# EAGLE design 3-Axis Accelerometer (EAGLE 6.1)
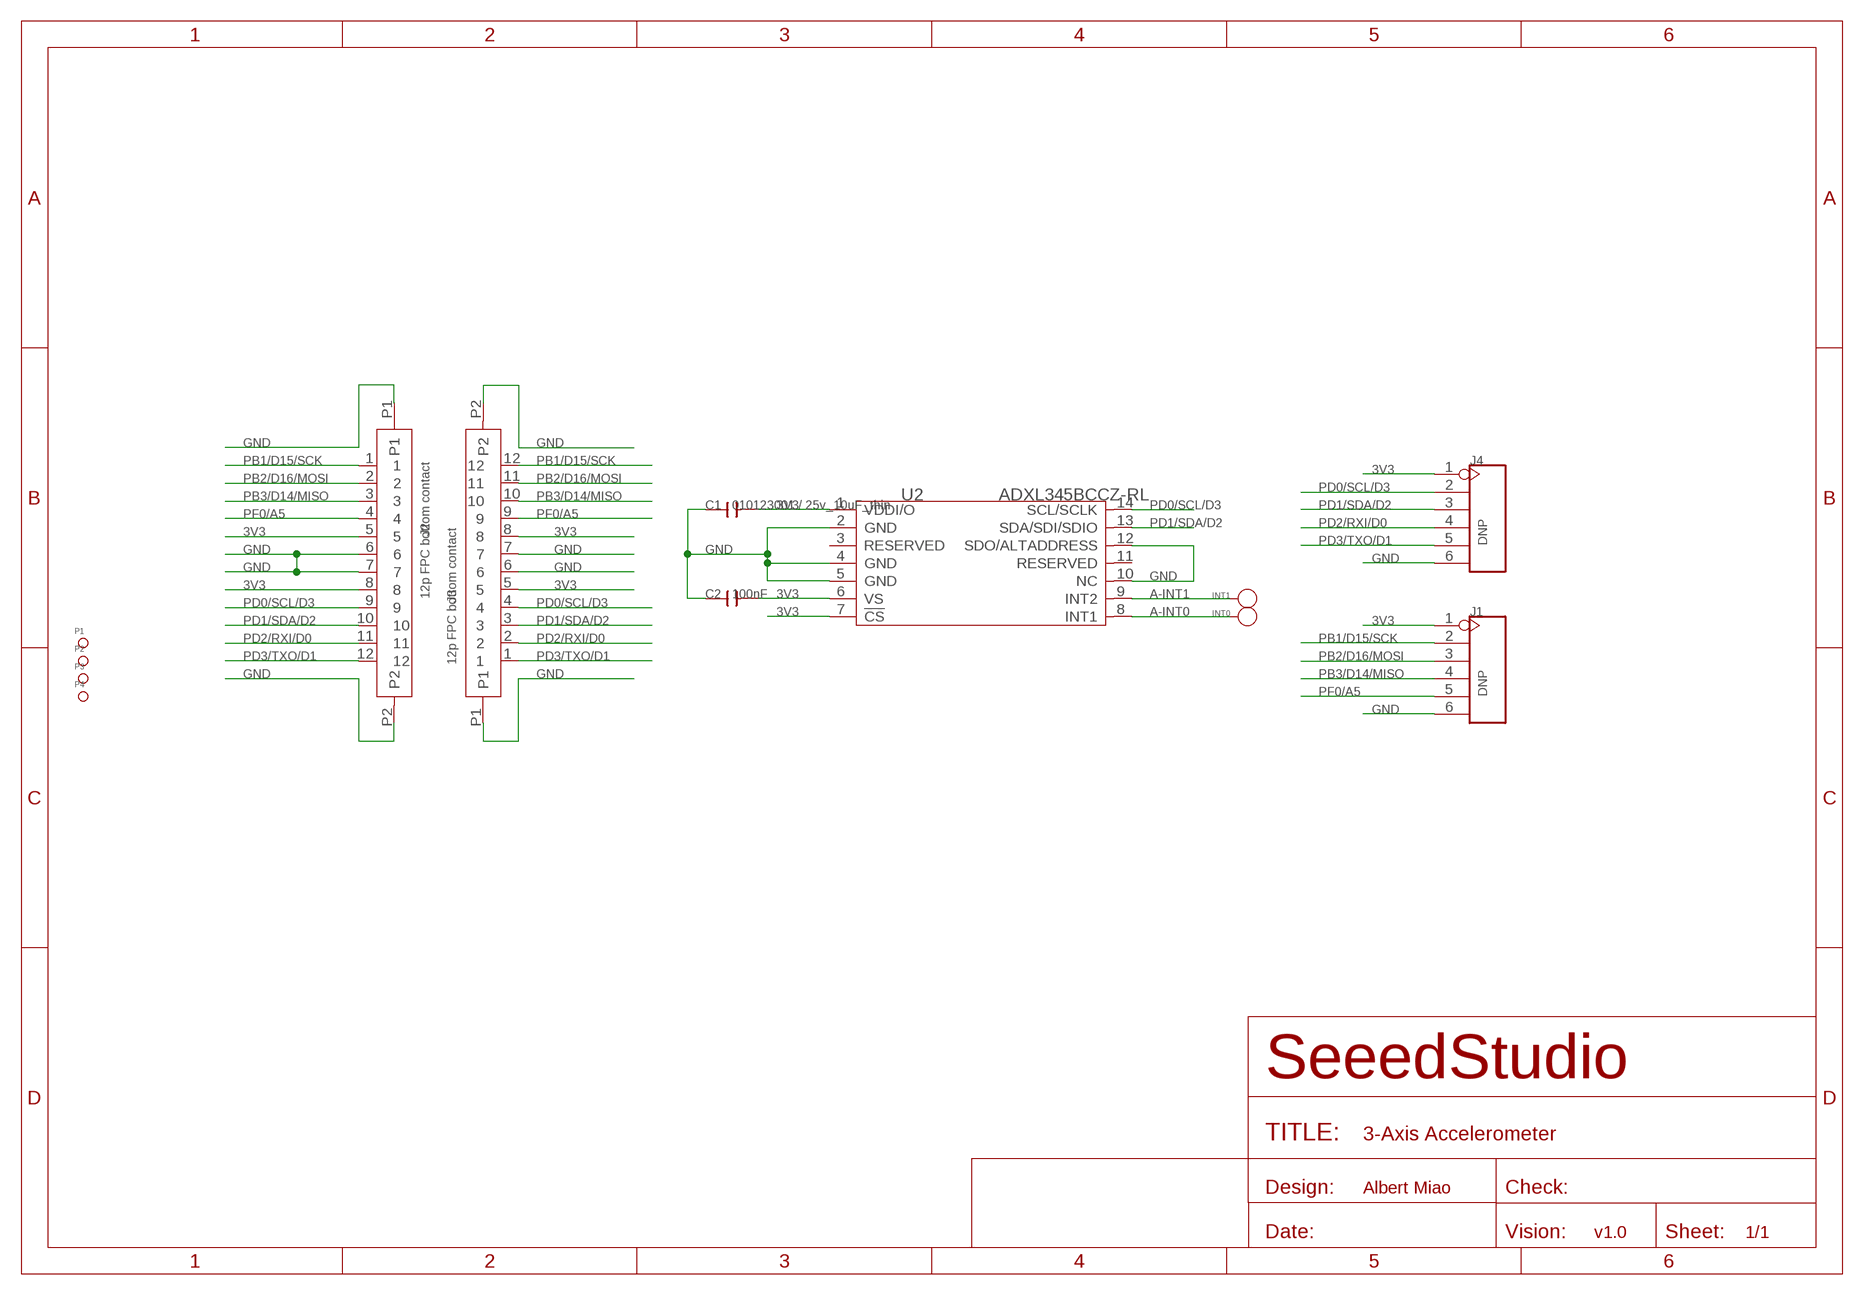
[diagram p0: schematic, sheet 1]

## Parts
C1  010123001 / 25v_10uF_thin  C-0805  [C0805]
C2  100nF  C-0603  [C0603]
INT0  DNP  PAD-TEST-POINT-CIRCLE'4545'  [TP_4545]
INT1  DNP  PAD-TEST-POINT-CIRCLE'4545'  [TP_4545]
J1  DNP  HEADER-6P-65/35MIL  [6P-2.54-65/35MIL]
J2  12p FPC bottom contact  FPC052002-12LT  [12P-0.5]
J3  12p FPC bottom contact  FPC052002-12LT  [12P-0.5]
J4  DNP  HEADER-6P-65/35MIL  [6P-2.54-65/35MIL]
P1  PAD-MARK  [ROUND-MARK-1.0]
P2  PAD-MARK  [ROUND-MARK-1.0]
P3  PAD-MARK  [ROUND-MARK-1.0]
P4  PAD-MARK  [ROUND-MARK-1.0]
U2  ADXL345BCCZ-RL  ADXL345  [LGA14]

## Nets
3V3: C1.2 C2.2 J1.1 J2.5 J2.8 J3.5 J3.8 J4.1 U2.1(VDDI/O) U2.6(VS) U2.7(!CS)
A-INT0: INT0.T U2.8(INT1)
A-INT1: INT1.T U2.9(INT2)
GND: C1.1 C2.1 J1.6 J2.6 J2.7 J2.P1 J2.P2 J3.6 J3.7 J3.P1 J3.P2 J4.6 U2.2(GND) U2.4(GND) U2.5(GND) U2.10(NC) U2.12(SDO/ALTADDRESS)
PB1/D15/SCK: J1.2 J2.1 J3.12
PB2/D16/MOSI: J1.3 J2.2 J3.11
PB3/D14/MISO: J1.4 J2.3 J3.10
PD0/SCL/D3: J2.9 J3.4 J4.2 U2.14(SCL/SCLK)
PD1/SDA/D2: J2.10 J3.3 J4.3 U2.13(SDA/SDI/SDIO)
PD2/RXI/D0: J2.11 J3.2 J4.4
PD3/TXO/D1: J2.12 J3.1 J4.5
PF0/A5: J1.5 J2.4 J3.9
Unconnected: U2.3(RESERVED) U2.11(RESERVED)

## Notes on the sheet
- Albert Miao
- v1.0

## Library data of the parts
C1 C2 = Discrete:C*: Ceramic Capacitors
INT0 INT1 = Discrete:PAD-TEST-POINT-CIRCLE; PARTNO: DNP
J1 J4 = Connector:HEADER-6P
J2 J3 = template:FPC052002-12LT
P1-P4 = Discrete:PAD-MARK; PARTNO: DNP
U2 = IC:ADXL345: 3-Axis,+/-2g / +/-4g / +/-8g / +/-16g Digital Accelerometer

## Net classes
0 default: width 0.152 mm, drill 0.305 mm, clearance 0.152 mm
1 GND: width 0.152 mm, drill 0.305 mm, clearance 0.152 mm to class 0, clearance 0.152 mm

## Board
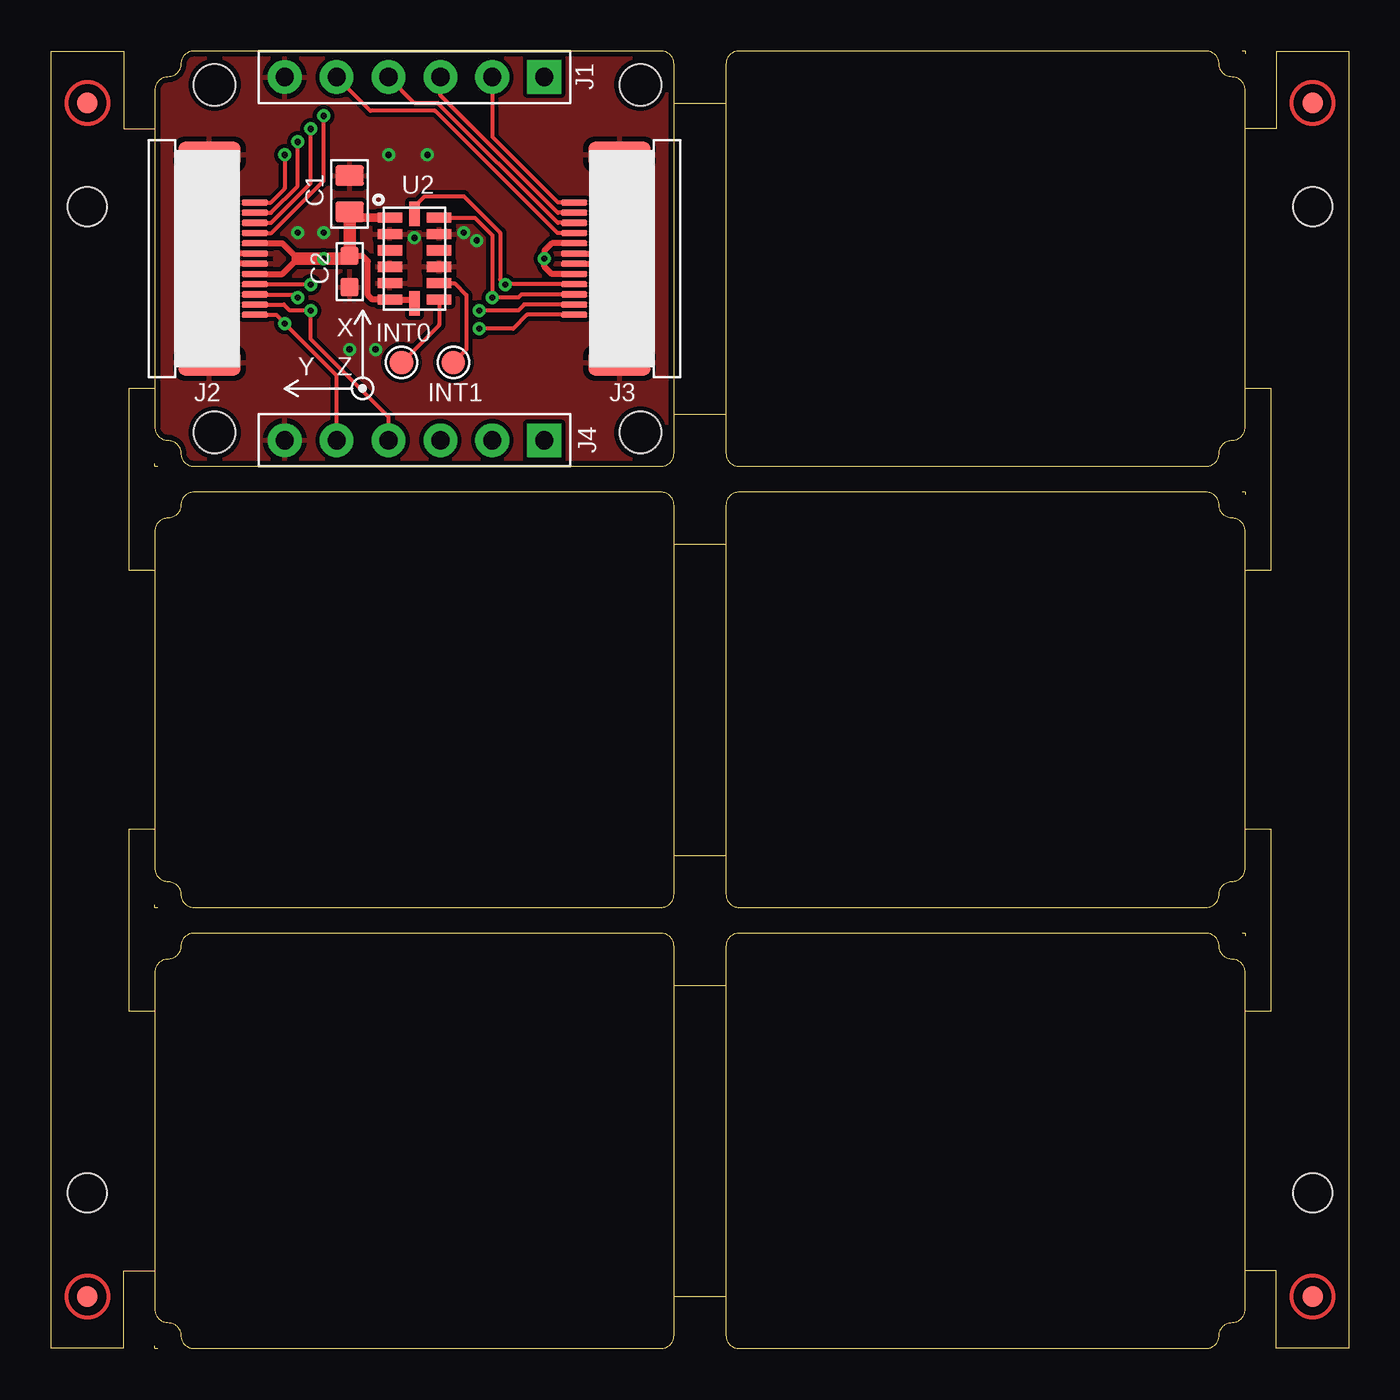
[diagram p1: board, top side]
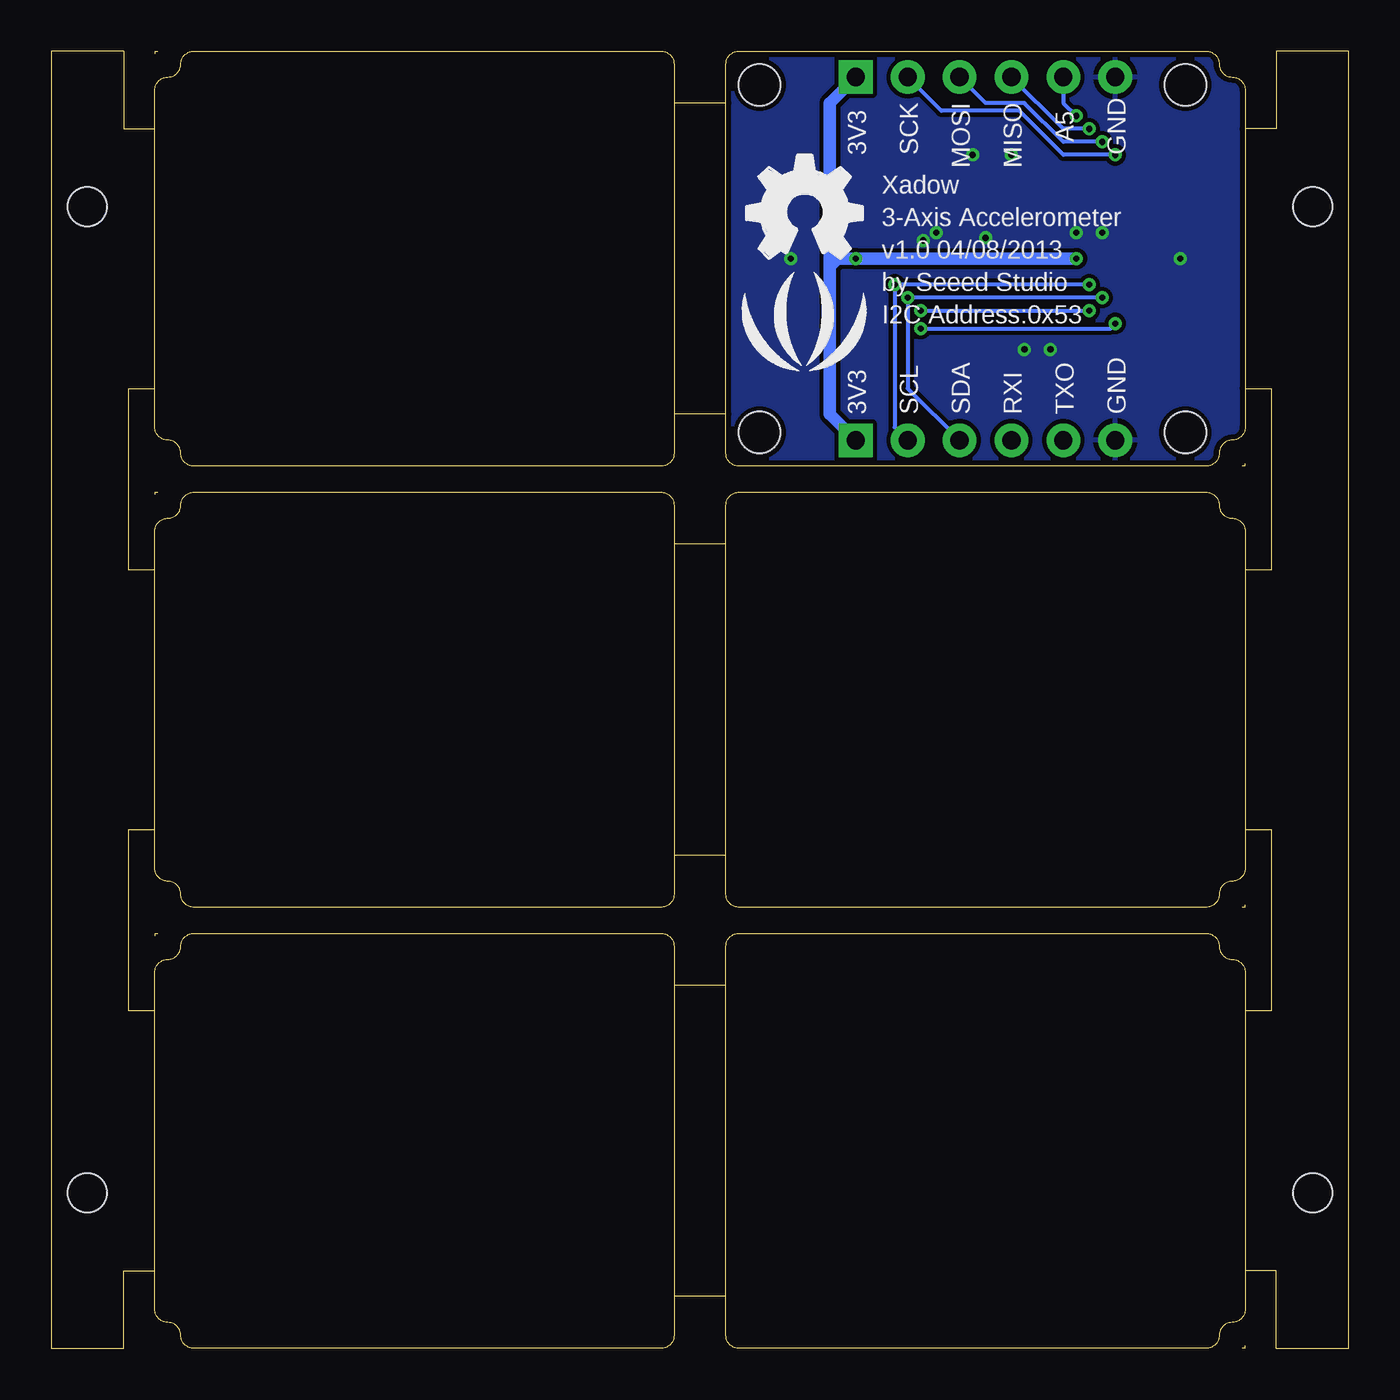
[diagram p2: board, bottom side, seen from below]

Size 63.5 x 63.5 mm. Coordinates in mm from the lower left corner, seen from the top.
Outline: 144 segments
Copper layers (1*16): Top 0.035mm / dielectric 1.5mm / Bottom 0.035mm
Design rules "SeeedStudio_rule_no_angle_090911 *": minimum track width 6mil, minimum drill 12mil, track to track 6mil, track to pad 6mil, pad to pad 6mil, via to via 6mil, smd to smd 0mil, copper to edge 10mil, drill to drill 10mil, minimum pad ring 10mil, minimum via ring 6mil, stop-mask expansion 2mil, vias tented up to drill 100mil, thermal gap 10mil
Holes 2.03 mm at 8,44.83 8,61.85 28.83,61.85 28.83,44.83
Holes 1.91 mm at 1.78,55.88 61.72,55.88 1.78,7.62 61.72,7.62
tRestrict: area 9.5,53.3 to 10.2,53.4; area 25.3,53.3 to 26,53.4; area 16.1,52.5 to 17.1,52.6; area 16.5,47.6 to 17.8,48.9; area 19.1,47.6 to 20.3,48.9; 13 lines
bRestrict: 13 lines

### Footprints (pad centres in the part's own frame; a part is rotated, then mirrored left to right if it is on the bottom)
C0805 = smd 1.016 x 1.397: 1 -0.889,0; 2 0.889,0
C0603 = smd 0.889 x 0.889: 1 -0.762,0; 2 0.762,0
TP_4545 = smd 1.143 x 1.143: T 0,0
6P-2.54-65/35MIL = drill 0.889 pad 1.651 square: 1 0,6.35 | drill 0.889 pad 1.651: 2 0,3.81; 3 0,1.27; 4 0,-1.27; 5 0,-3.81; 6 0,-6.35
12P-0.5 = smd 0.3 x 1.3: 1 -2.75,2.35; 2 -2.25,2.35; 3 -1.75,2.35; 4 -1.25,2.35; 5 -0.75,2.35; 6 -0.25,2.35; 7 0.25,2.35; 8 0.75,2.35; 9 1.25,2.35; 10 1.75,2.35; 11 2.25,2.35; 12 2.75,2.35 | smd 1.27 x 3.048: P1 -5.08,0.127; P2 5.08,0.127
ROUND-MARK-1.0 = smd 1.016 x 1.016: P$1 0,0
LGA14 = smd 1.2 x 0.5: 1 -1.2,2; 2 -1.2,1.2; 3 -1.2,0.4; 4 -1.2,-0.4; 5 -1.2,-1.2; 6 -1.2,-2; 8 1.2,-2; 9 1.2,-1.2; 10 1.2,-0.4; 11 1.2,0.4; 12 1.2,1.2; 13 1.2,2 | smd 0.5 x 1.2: 7 0,-2.2; 14 0,2.2

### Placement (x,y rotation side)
C1  14.61,56.52 270 top
C2  14.61,52.71 90 top
INT0  17.14,48.26 0 top
INT1  19.69,48.26 0 top
J1  17.78,62.23 270 top
J2  7.62,53.34 270 top
J3  27.94,53.34 90 top
J4  17.78,44.45 270 top
P1  1.78,60.96 180 top
P2  1.78,2.54 0 top
P3  61.72,2.54 0 top
P4  61.72,60.96 0 top
U2  17.78,53.34 0 top
U$2  [LOGO_SILK]  26.67,49.53 0 bottom
U$3  [OSHW_FILLX200_NOTEXT]  29.46,53.34 0 bottom

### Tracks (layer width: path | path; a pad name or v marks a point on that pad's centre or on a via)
3V3  (via drill 0.3 pad 0.64)
  Top 0.305: J2.5 11.32,54.09 12.07,53.34 11.32,52.59 J2.8 | J3.5 24.5,52.59 24.13,52.96 v24.13,53.34 24.13,53.72 24.5,54.09 J3.8 | U2.7 17.58,51.34 U2.6 15.72,51.34 15.49,51.56 15.49,53.21 15.24,53.47 C2.2
  Top 0.406: U2.1 14.89,55.34 C1.2
  Top 0.61: 12.07,53.34 v13.34,53.34 14.48,53.34 C2.2 C1.2
  Bottom 0.61: J1.1 25.4,60.96 25.4,53.72 | 25.4,53.72 25.4,52.96 | 25.4,52.96 25.4,45.72 J4.1 | 25.02,53.34 v24.13,53.34 v13.34,53.34 | 25.02,53.34 25.4,53.72 | 25.4,52.96 25.02,53.34
A-INT0
  Top 0.203: U2.8 18.98,50.1 INT0.T
A-INT1
  Top 0.203: U2.9 19.74,52.14 20.32,51.56 20.32,48.9 INT1.T
GND  (via drill 0.3 pad 0.64)
  Top 0.305: J2.6 8.51,53.59 8.32,53.4 | 8.32,53.4 v8.26,53.34 | J2.7 8.63,53.09 8.32,53.4 | J3.7 27.05,53.59 v27.3,53.34 27.05,53.09 J3.6
  other vias: 17.78,54.36 12.07,54.61 13.34,54.61 14.61,48.9 15.88,48.9 16.51,58.42 18.42,58.42 20.83,54.23 20.19,54.61
  pour Top (isolate 0.203): 5.08,43.18 30.48,43.18 30.48,63.5 5.08,63.5 5.08,43.31
  pour Bottom (isolate 0.203): 5.08,43.18 30.48,43.18 30.48,63.5 5.08,63.5 5.08,43.31
PB1/D15/SCK  (via drill 0.3 pad 0.64)
  Top 0.203: J1.2 21.59,59.31 24.81,56.09 J3.12 | v11.43,58.42 11.43,56.77 10.75,56.09 J2.1
  Bottom 0.203: v11.43,58.42 13.97,58.42 16.13,60.58 19.94,60.58 J1.2
PB2/D16/MOSI  (via drill 0.3 pad 0.64)
  Top 0.203: J3.11 24.8,55.59 19.05,61.34 J1.3 | J2.2 10.76,55.59 12.07,56.9 v12.07,59.06
  Bottom 0.203: v12.07,59.06 13.97,59.06 15.88,60.96 17.78,60.96 J1.3
PB3/D14/MISO  (via drill 0.3 pad 0.64)
  Top 0.203: J3.10 24.79,55.09 18.92,60.96 17.78,60.96 J1.4 | J2.3 10.77,55.09 12.7,57.02 v12.7,59.69
  Bottom 0.203: v12.7,59.69 13.97,59.69 J1.4
PD0/SCL/D3  (via drill 0.3 pad 0.64)
  Top 0.203: U2.14 17.78,55.88 18.29,56.39 20.19,56.39 21.97,54.61 21.97,52.32 v22.23,52.07 22.25,52.09 J3.4 | J2.9 12.68,52.09 v12.7,52.07
  Bottom 0.203: v12.7,52.07 v22.23,52.07 22.23,45.09 J4.2
PD1/SDA/D2  (via drill 0.3 pad 0.64)
  Top 0.203: U2.13 20.73,55.34 21.59,54.48 v21.59,51.44 22.86,51.44 23.02,51.59 J3.3 | J2.10 11.91,51.59 v12.07,51.44
  Bottom 0.203: v12.07,51.44 v21.59,51.44 21.59,46.99 J4.3
PD2/RXI/D0  (via drill 0.3 pad 0.64)
  Top 0.203: J3.2 23.15,51.09 22.86,50.8 v20.96,50.8 | J2.11 11.39,51.09 11.68,50.8 v12.7,50.8 12.7,49.4 16.51,45.59 J4.4
  Bottom 0.203: v20.96,50.8 v12.7,50.8
PD3/TXO/D1  (via drill 0.3 pad 0.64)
  Top 0.203: J3.1 23.29,50.59 22.61,49.91 v20.96,49.91 | J2.12 11.01,50.59 v11.43,50.17 13.97,47.63 J4.5
  Bottom 0.203: v20.96,49.91 11.68,49.91 v11.43,50.17
PF0/A5  (via drill 0.3 pad 0.64)
  Top 0.203: J3.9 24.79,54.59 18.8,60.58 15.62,60.58 J1.5 | J2.4 10.78,54.59 13.34,57.15 v13.34,60.33
  Bottom 0.203: J1.5 13.97,60.96 v13.34,60.33

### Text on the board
tPlace: X | Y | Z
bPlace: A5 | GND | SCK | 3V3 | MISO | MOSI | Xadow | 3-Axis Accelerometer | v1.0 04/08/2013 | by Seeed Studio | I2C Address:0x53 | GND | TXO | RXI | SDA | SCL | 3V3
tEnhance: Top Enhance 0.25~0.28mm
bEnhance: Bottom Enhance
bEnHoles: Holes on Bottom Enhance | All Holes are 70mil diameter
